| IBIS file stm32l552_562_lqfp64.ibs
[IBIS ver]   4.2
[File name]  stm32l552_562_lqfp64.ibs
[File Rev]   1.0
[Date]   04-10-2019
[Source]   Data Created at STMicroelectronics
[Notes]   File originated from ELDO simulations.
[Disclaimer] This information is for modeling purpose only and is
   not guaranted.
   The information is subject to change without notice.
[Copyright]  Copyright 2019 STMicroelectronics Inc.
|   Component stm32l552_562_lqfp64
[Component] stm32l552_562_lqfp64
[Manufacturer] STMicroelectronics
[Package]
| variable   typ   min   max
R_pkg  0  NA  NA
L_pkg  0  NA  NA
C_pkg  0  NA  NA
[Pin]   signal_name   model_name R_pin L_pin C_pin
1 VBAT POWER 68.980E-3 4.220E-9 120.000E-15
2 PC13 io8prog2m25m50m120m_sudq_ft 63.756E-3 3.679E-9 93.469E-15
3 PC14-OSC32_IN io8prog2m25m50m120m_sudq_ft 59.336E-3 3.221E-9 71.020E-15
4 PC15-OSC32_OUT io8prog2m25m50m120m_sudq_ft 55.719E-3 2.846E-9 52.653E-15
5 PH0-OSC_IN io8prog2m25m50m120m_sudq_ft 52.907E-3 2.555E-9 38.367E-15
6 PH1-OSC_OUT io8prog2m25m50m120m_sudq_ft 50.897E-3 2.347E-9 28.163E-15
7 NRST ioreset_ft_v33 49.692E-3 2.222E-9 22.041E-15
8 PC0 io8prog2m25m50m120m_sudq_i2c_ft 49.290E-3 2.180E-9 20.000E-15
9 PC1 io8prog2m25m50m120m_sudq_i2c_ft 49.290E-3 2.180E-9 20.000E-15
10 PC2 io8prog2m25m50m120m_sudq_ft 49.692E-3 2.222E-9 22.041E-15
11 PC3 io8prog2m25m50m120m_sudq_ft 50.897E-3 2.347E-9 28.163E-15
12 VSSA_VREF- GND 52.907E-3 2.555E-9 38.367E-15
13 VDDA_VREF+ POWER 55.719E-3 2.846E-9 52.653E-15
14 PA0 io8prog2m25m50m120m_sudq_ft 59.336E-3 3.221E-9 71.020E-15
15 PA1 io8prog2m25m50m120m_sudq_ft 63.756E-3 3.679E-9 93.469E-15
16 PA2 io8prog2m25m50m120m_sudq_ft 68.980E-3 4.220E-9 120.000E-15
17 PA3 io8prog2m25m50m120m_sudq_ft 68.980E-3 4.220E-9 120.000E-15
18 VSS GND 63.756E-3 3.679E-9 93.469E-15
19 VDD POWER 59.336E-3 3.221E-9 71.020E-15
20 PA4 io8prog2m25m50m120m_sudq_ft 55.719E-3 2.846E-9 52.653E-15
21 PA5 io8prog2m25m50m120m_sudq_ft 52.907E-3 2.555E-9 38.367E-15
22 PA6 io8prog2m25m50m120m_sudq_ft 50.897E-3 2.347E-9 28.163E-15
23 PA7 io8prog2m25m50m120m_sudq_i2c_ft 49.692E-3 2.222E-9 22.041E-15
24 PC4 io8prog2m25m50m120m_sudq_ft 49.290E-3 2.180E-9 20.000E-15
25 PC5 io8prog2m25m50m120m_sudq_ft 49.290E-3 2.180E-9 20.000E-15
26 PB0 io8prog2m25m50m120m_sudq_ft 49.692E-3 2.222E-9 22.041E-15
27 PB1 io8prog2m25m50m120m_sudq_ft 50.897E-3 2.347E-9 28.163E-15
28 PB2 io8prog2m25m50m120m_sudq_ft 52.907E-3 2.555E-9 38.367E-15
29 PB10 io8prog2m25m50m120m_sudq_i2c_ft 55.719E-3 2.846E-9 52.653E-15
30 PB11 io8prog2m25m50m120m_sudq_i2c_ft 59.336E-3 3.221E-9 71.020E-15
31 VSS GND 63.756E-3 3.679E-9 93.469E-15
32 VDD POWER 68.980E-3 4.220E-9 120.000E-15
33 PB12 io8prog2m25m50m120m_sudq_ft 68.980E-3 4.220E-9 120.000E-15
34 PB13 io8prog2m25m50m120m_sudq_i2c_ft 63.756E-3 3.679E-9 93.469E-15
35 PB14 io8prog2m25m50m120m_sudq_i2c_ft 59.336E-3 3.221E-9 71.020E-15
36 PB15 io6usb_bmc_pd_cc_ft 55.719E-3 2.846E-9 52.653E-15
37 PC6 io8prog2m25m50m120m_sudq_ft 52.907E-3 2.555E-9 38.367E-15
38 PC7 io8prog2m25m50m120m_sudq_ft 50.897E-3 2.347E-9 28.163E-15
39 PC8 io8prog2m25m50m120m_sudq_ft 49.692E-3 2.222E-9 22.041E-15
40 PC9 io8prog2m25m50m120m_sudq_i2c_ft 49.290E-3 2.180E-9 20.000E-15
41 PA8 io8prog2m25m50m120m_sudq_i2c_ft 49.290E-3 2.180E-9 20.000E-15
42 PA9 io8prog2m25m50m120m_sudq_ft 49.692E-3 2.222E-9 22.041E-15
43 PA10 io8prog2m25m50m120m_sudq_ft 50.897E-3 2.347E-9 28.163E-15
44 PA11 io8usblsfs_otg2 52.907E-3 2.555E-9 38.367E-15
45 PA12 io8usblsfs_otg2 55.719E-3 2.846E-9 52.653E-15
46 PA13 io8prog2m25m50m120m_sudq_ft 59.336E-3 3.221E-9 71.020E-15
47 VSS GND 63.756E-3 3.679E-9 93.469E-15
48 VDDUSB POWER 68.980E-3 4.220E-9 120.000E-15
49 PA14 io8prog2m25m50m120m_sudq_i2c_ft 68.980E-3 4.220E-9 120.000E-15
50 PA15 io6usb_bmc_pd_cc_ft 63.756E-3 3.679E-9 93.469E-15
51 PC10 io8prog2m25m50m120m_sudq_ft 59.336E-3 3.221E-9 71.020E-15
52 PC11 io8prog2m25m50m120m_sudq_ft 55.719E-3 2.846E-9 52.653E-15
53 PC12 io8prog2m25m50m120m_sudq_ft 52.907E-3 2.555E-9 38.367E-15
54 PD2 io8prog2m25m50m120m_sudq_ft 50.897E-3 2.347E-9 28.163E-15
55 PB3 io8prog2m25m50m120m_sudq_ft 49.692E-3 2.222E-9 22.041E-15
56 PB4 io8prog2m25m50m120m_sudq_i2c_ft 49.290E-3 2.180E-9 20.000E-15
57 PB5 io8prog2m25m50m120m_sudq_ft 49.290E-3 2.180E-9 20.000E-15
58 PB6 io8prog2m25m50m120m_sudq_i2c_ft 49.692E-3 2.222E-9 22.041E-15
59 PB7 io8prog2m25m50m120m_sudq_i2c_ft 50.897E-3 2.347E-9 28.163E-15
60 PH3-BOOT0 io8prog2m25m50m120m_sudq_ft 52.907E-3 2.555E-9 38.367E-15
61 PB8 io8prog2m25m50m120m_sudq_i2c_ft 55.719E-3 2.846E-9 52.653E-15
62 PB9 io8prog2m25m50m120m_sudq_i2c_ft 59.336E-3 3.221E-9 71.020E-15
63 VSS GND 63.756E-3 3.679E-9 93.469E-15
64 VDD POWER 68.980E-3 4.220E-9 120.000E-15
[Model Selector] io6usb_bmc_pd_cc_ft
usb_bmc_emit_pdccpd  "BMC PD emitter  + PD"
usb_bmc_emit_pdcc3a0  "BMC PD emitter  + 3rd PU"
usb_bmc_emit_pdcc1a5  "BMC PD emitter  + 2nd PU"
usb_bmc_emit_pdccusb  "BMC PD emitter  + 1st PU"
usb_bmc_emit  "BMC PD emitter "
io2_pdcc_ft_3v3_lowspeed  "GPIO-3.3V range - low speed"
io2_pdcc_ft_3v3_mediumspeed  "GPIO-3.3V range - medium speed"
io2_pdcc_ft_3v3_lowspeed_pu  "GPIO-3.3V range - low speed - pull up"
io2_pdcc_ft_3v3_mediumspeed_pu  "GPIO-3.3V range - medium speed - pull up"
io2_pdcc_ft_3v3_lowspeed_pd  "GPIO-3.3V range - low speed - pull down"
io2_pdcc_ft_3v3_mediumspeed_pd  "GPIO-3.3V range - medium speed - pull down"
io2_pdcc_ft_1v8_lowspeed  "GPIO-1.8V range - low speed"
io2_pdcc_ft_1v8_mediumspeed  "GPIO-1.8V range - medium speed"
io2_pdcc_ft_1v8_lowspeed_pu  "GPIO-1.8V range - low speed - pull up"
io2_pdcc_ft_1v8_mediumspeed_pu  "GPIO-1.8V range - medium speed - pull up"
io2_pdcc_ft_1v8_lowspeed_pd  "GPIO-1.8V range - low speed - pull down"
io2_pdcc_ft_1v8_mediumspeed_pd  "GPIO-1.8V range - medium speed - pull down"
io2_pdcc_ft_1v2_lowspeed  "GPIO-1.2V range - low speed"
io2_pdcc_ft_1v2_mediumspeed  "GPIO-1.2V range - medium speed"
io2_pdcc_ft_1v2_lowspeed_pu  "GPIO-1.2V range - low speed - pull up"
io2_pdcc_ft_1v2_mediumspeed_pu  "GPIO-1.2V range - medium speed - pull up"
io2_pdcc_ft_1v2_lowspeed_pd  "GPIO-1.2V range - low speed - pull down"
io2_pdcc_ft_1v2_mediumspeed_pd  "GPIO-1.2V range - medium speed - pull down"
[Model Selector] io8prog2m25m50m120m_sudq_ft
iols8p_sudq_ft_pd_lv  "IO low speed, PD=40kOhm - 1P8V"
iols8p_sudq_ft_pu_lv  "IO low speed, PU=40kOhm - 1P8V"
iols8p_sudq_ft_lv  "IO low speed - 1P8V"
iols8p_sudq_ft_pd  "IO low speed, PD=40kOhm - 3P3V"
iols8p_sudq_ft_pu  "IO low speed, PU=40kOhm - 3P3V"
iols8p_sudq_ft  "IO low speed - 3P3V"
iofs8p_sudq_ft_pd_lv  "IO full speed, PD=40kOhm - 1P8V"
iofs8p_sudq_ft_pu_lv  "IO full speed, PU=40kOhm - 1P8V"
iofs8p_sudq_ft_lv  "IO full speed - 1P8V"
iofs8p_sudq_ft_pd  "IO full speed, PD=40kOhm - 3P3V"
iofs8p_sudq_ft_pu  "IO full speed, PU=40kOhm - 3P3V"
iofs8p_sudq_ft  "IO full speed - 3P3V"
ioms8p_sudq_ft_pd_lv  "IO medium speed, PD=40kOhm - 1P8V"
ioms8p_sudq_ft_pu_lv  "IO medium speed, PU=40kOhm - 1P8V"
ioms8p_sudq_ft_lv  "IO medium speed - 1P8V"
ioms8p_sudq_ft_pd  "IO medium speed, PD=40kOhm - 3P3V"
ioms8p_sudq_ft_pu  "IO medium speed, PU=40kOhm - 3P3V"
ioms8p_sudq_ft  "IO medium speed - 3P3V"
iohs8p_sudq_ft_pd_lv  "IO high speed, PD=40kOhm - 1P8V"
iohs8p_sudq_ft_pu_lv  "IO high speed, PU=40kOhm - 1P8V"
iohs8p_sudq_ft_lv  "IO high speed - 1P8V"
iohs8p_sudq_ft_pd  "IO high speed, PD=40kOhm - 3P3V"
iohs8p_sudq_ft_pu  "IO high speed, PU=40kOhm - 3P3V"
iohs8p_sudq_ft  "IO high speed - 3P3V"
[Model Selector] io8prog2m25m50m120m_sudq_i2c_ft
io8prog_1v8_i2c_pd  "5V Tol GPIO 1.8V range i2c functionality with pull down"
io8prog_1v8_i2c_pu  "5V Tol GPIO 1.8V range i2c functionality with pull up"
io8prog_1v8_i2c  "5V Tol GPIO 1.8V range i2c functionality"
io8prog_3v3_i2c_pd  "5V Tol GPIO 3.3V range i2c functionality with pull down"
io8prog_3v3_i2c_pu  "5V Tol GPIO 3.3V range i2c functionality with pull up"
io8prog_3v3_i2c  "5V Tol GPIO 3.3V range i2c functionality"
iols8p_sudq_ft_pd_lv  "IO low speed, PD=40kOhm - 1P8V"
iols8p_sudq_ft_pu_lv  "IO low speed, PU=40kOhm - 1P8V"
iols8p_sudq_ft_lv  "IO low speed - 1P8V"
iols8p_sudq_ft_pd  "IO low speed, PD=40kOhm - 3P3V"
iols8p_sudq_ft_pu  "IO low speed, PU=40kOhm - 3P3V"
iols8p_sudq_ft  "IO low speed - 3P3V"
iofs8p_sudq_ft_pd_lv  "IO full speed, PD=40kOhm - 1P8V"
iofs8p_sudq_ft_pu_lv  "IO full speed, PU=40kOhm - 1P8V"
iofs8p_sudq_ft_lv  "IO full speed - 1P8V"
iofs8p_sudq_ft_pd  "IO full speed, PD=40kOhm - 3P3V"
iofs8p_sudq_ft_pu  "IO full speed, PU=40kOhm - 3P3V"
iofs8p_sudq_ft  "IO full speed - 3P3V"
ioms8p_sudq_ft_pd_lv  "IO medium speed, PD=40kOhm - 1P8V"
ioms8p_sudq_ft_pu_lv  "IO medium speed, PU=40kOhm - 1P8V"
ioms8p_sudq_ft_lv  "IO medium speed - 1P8V"
ioms8p_sudq_ft_pd  "IO medium speed, PD=40kOhm - 3P3V"
ioms8p_sudq_ft_pu  "IO medium speed, PU=40kOhm - 3P3V"
ioms8p_sudq_ft  "IO medium speed - 3P3V"
iohs8p_sudq_ft_pd_lv  "IO high speed, PD=40kOhm - 1P8V"
iohs8p_sudq_ft_pu_lv  "IO high speed, PU=40kOhm - 1P8V"
iohs8p_sudq_ft_lv  "IO high speed - 1P8V"
iohs8p_sudq_ft_pd  "IO high speed, PD=40kOhm - 3P3V"
iohs8p_sudq_ft_pu  "IO high speed, PU=40kOhm - 3P3V"
iohs8p_sudq_ft  "IO high speed - 3P3V"
[Model Selector] io8usblsfs_otg2
usb_ls_pd  "USB Low Speed mode - Pull Down"
usb_ls_pu2  "USB Low Speed mode - Pull up 2"
usb_ls_pu  "USB Low Speed mode - Pull up"
usb_fs  "USB Low Speed mode"
usb_fs_pd  "USB Full Speed mode - Pull Down"
usb_fs_pu2  "USB Full Speed mode - Pull up 2"
usb_fs_pu  "USB Full Speed mode - Pull up"
[Model Selector] ioreset_ft_v33
ioreset_1v2_pu  "RESET 1.2V range with PU"
ioreset_1v2  "RESET 1.2V range"
ioreset_1v8_pu  "RESET 1.8V range with PU"
ioreset_1v8  "RESET 1.8V range"
ioreset_3v3_pu  "RESET 3.3V range with PU"
ioreset_3v3  "RESET 3.3V range"
| Models and submodels in the file (66): usb_bmc_emit_pdccpd (I/O), usb_bmc_emit_pdcc3a0 (I/O), usb_bmc_emit_pdcc1a5 (I/O), usb_bmc_emit_pdccusb (I/O), usb_bmc_emit (I/O), io2_pdcc_ft_3v3_lowspeed (I/O), io2_pdcc_ft_3v3_mediumspeed (I/O), io2_pdcc_ft_3v3_lowspeed_pu (I/O), io2_pdcc_ft_3v3_mediumspeed_pu (I/O), io2_pdcc_ft_3v3_lowspeed_pd (I/O), io2_pdcc_ft_3v3_mediumspeed_pd (I/O), io2_pdcc_ft_1v8_lowspeed (I/O), io2_pdcc_ft_1v8_mediumspeed (I/O), io2_pdcc_ft_1v8_lowspeed_pu (I/O), io2_pdcc_ft_1v8_mediumspeed_pu (I/O), io2_pdcc_ft_1v8_lowspeed_pd (I/O), io2_pdcc_ft_1v8_mediumspeed_pd (I/O), io2_pdcc_ft_1v2_lowspeed (I/O), io2_pdcc_ft_1v2_mediumspeed (I/O), io2_pdcc_ft_1v2_lowspeed_pu (I/O), io2_pdcc_ft_1v2_mediumspeed_pu (I/O), io2_pdcc_ft_1v2_lowspeed_pd (I/O), io2_pdcc_ft_1v2_mediumspeed_pd (I/O), iols8p_sudq_ft_pd_lv (I/O), iols8p_sudq_ft_pu_lv (I/O), iols8p_sudq_ft_lv (I/O), iols8p_sudq_ft_pd (I/O), iols8p_sudq_ft_pu (I/O), iols8p_sudq_ft (I/O), iofs8p_sudq_ft_pd_lv (I/O), iofs8p_sudq_ft_pu_lv (I/O), iofs8p_sudq_ft_lv (I/O), iofs8p_sudq_ft_pd (I/O), iofs8p_sudq_ft_pu (I/O), iofs8p_sudq_ft (I/O), ioms8p_sudq_ft_pd_lv (I/O), ioms8p_sudq_ft_pu_lv (I/O), ioms8p_sudq_ft_lv (I/O), ioms8p_sudq_ft_pd (I/O), ioms8p_sudq_ft_pu (I/O), ioms8p_sudq_ft (I/O), iohs8p_sudq_ft_pd_lv (I/O), iohs8p_sudq_ft_pu_lv (I/O), iohs8p_sudq_ft_lv (I/O), iohs8p_sudq_ft_pd (I/O), iohs8p_sudq_ft_pu (I/O), iohs8p_sudq_ft (I/O), io8prog_1v8_i2c_pd (I/O_open_drain), io8prog_1v8_i2c_pu (I/O_open_drain), io8prog_1v8_i2c (I/O_open_drain), io8prog_3v3_i2c_pd (I/O_open_drain), io8prog_3v3_i2c_pu (I/O_open_drain), io8prog_3v3_i2c (I/O_open_drain), usb_ls_pd (I/O), usb_ls_pu2 (I/O), usb_ls_pu (I/O), usb_fs (I/O), usb_fs_pd (I/O), usb_fs_pu2 (I/O), usb_fs_pu (I/O), ioreset_1v2_pu (I/O_open_drain), ioreset_1v2 (I/O_open_drain), ioreset_1v8_pu (I/O_open_drain), ioreset_1v8 (I/O_open_drain), ioreset_3v3_pu (I/O_open_drain), ioreset_3v3 (I/O_open_drain)
